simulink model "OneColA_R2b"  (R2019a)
settings: Solver=ode15s  StartTime=0.0  StopTime=tend  RelTol=1e-3
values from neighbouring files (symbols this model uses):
  alpha_L = -abs(alpha(2))    [TuningSRC.m]
  alpha_V = abs(alpha(1))    [TuningSRC.m]
  biasL = 3.2    [TuningSRC.m]
  biasV = VB0    [TuningSRC.m]
  DeltaxDmin = -0.01    [Simulate1Col_R2.m]
  Extract_J = zeros(83,1)'    [Simulate1Col.m]    (also in Simulate1Col_OL.m; Simulate1Col_R1.m; Simulate1Col_R2.m)
  Extract_xB = zeros(82,1)'    [Simulate1Col.m]    (also in Simulate1Col_OL.m; Simulate1Col_R1.m; Simulate1Col_R2.m)
  Extract_xD = zeros(82,1)'    [Simulate1Col.m]    (also in Simulate1Col_OL.m; Simulate1Col_R1.m; Simulate1Col_R2.m)
  F0 = 1    [colamod.m]    (also in ColumnA_simulation.m; Simulate1Col.m = F; Simulate1Col_OL.m = F; Simulate1Col_R1.m = F)
  F0step = 0.05    [Simulate1Col.m]    (also in Simulate1Col_OL.m = 1*F0*.1; Simulate1Col_R1.m; Simulate1Col_R2.m = 0.15)
  F0step2 = 0*(0.15-F0step)    (= 0)    [Simulate1Col.m]    (also in Simulate1Col_R1.m; Simulate1Col_R2.m = 0.1)
  F0step2_t = 30    [Simulate1Col.m]    (also in Simulate1Col_R1.m; Simulate1Col_R2.m = 80)
  F0step3 = 0    [Simulate1Col_R2.m]
  F0step3_t = 180    [Simulate1Col_R2.m]
  F0step_t = 10    [Simulate1Col.m]    (also in Simulate1Col_OL.m; Simulate1Col_R1.m; Simulate1Col_R2.m)
  Fbias = Fmax    (= 1.6825)    [Simulate1Col_R2.m]
  Fmax = 1.6825    [Simulate1Col_R2.m]
  Jcol = pf*u_all(5) + pV*u_all(2) - pB*u_all(4) - pD*u_all(3)    [ColumnA_simulation.m]    (also in col_obj.m = pf*F + pV*V - pB*B - pD*D; LVMassBalance.m = pf*Feed + pV*Steam - pB*B - pD*D)
  Kc_FxD = tau_FxD /(K_FxD *(tauc_FxD+theta_FxD))    (= -1.50442477876)    [TuningCol.m]
  Kc_LTxD = tau_LTxD /(K_LTxD *(tauc_LTxD+theta_LTxD))    (= 23.0752764867)    [TuningCol.m]
  Kc_SRC = abs(Kc_SRC)    [TuningSRC.m]
  KI_FxD = Kc_FxD/tauI_FxD    [TuningCol.m]
  KI_LTxD = Kc_LTxD/tauI_LTxD    [TuningCol.m]
  KI_SRC = Kc_SRC/tauI_SRC    [TuningSRC.m]
  LmaxPI = Lmax-LT0    [Simulate1Col.m]    (also in Simulate1Col_R1.m; Simulate1Col_R2.m)
  LT0 = u_opt(1)    [Simulate1Col.m]    (also in Simulate1Col_OL.m; Simulate1Col_R1.m; Simulate1Col_R2.m)
  pV0 = pV    [Simulate1Col.m]    (also in Simulate1Col_OL.m; Simulate1Col_R1.m; Simulate1Col_R2.m)
  pVstep = 0.02    [Simulate1Col.m]    (also in Simulate1Col_OL.m = 0*(0.13-pV0); Simulate1Col_R1.m; Simulate1Col_R2.m = 0.06)
  pVstep2 = 0    [Simulate1Col_R2.m]
  pVstep2t = 140    [Simulate1Col_R2.m]
  pVstept = 50    [Simulate1Col.m]    (also in Simulate1Col_OL.m; Simulate1Col_R1.m; Simulate1Col_R2.m)
  qF = U(7)    [colamod.m]    (also in ColumnA_simulation.m; Simulate1Col.m = 1; Simulate1Col_OL.m = 1; Simulate1Col_R1.m = 1)
  tauI_SRC = (tauI_VxB+tauI_LTxB)/2    [TuningSRC.m]
  VB0 = u_opt(2)    [Simulate1Col.m]    (also in Simulate1Col_OL.m; Simulate1Col_R1.m; Simulate1Col_R2.m)
  Vmax = 4    [Simulate1Col.m]    (also in Simulate1Col_R1.m; Simulate1Col_R2.m; TuningSRC.m)
  x0 = 0.5*ones(1,82)'    [col_obj.m]    (also in Simulate1Col.m = x; Simulate1Col_OL.m = x; Simulate1Col_R1.m = x; Simulate1Col_R2.m = x)
  xBsp = 0.95    [Simulate1Col.m]    (also in Simulate1Col_OL.m; Simulate1Col_R1.m; Simulate1Col_R2.m)
  xDmin = 0.95    [Simulate1Col.m]    (also in Simulate1Col_OL.m; Simulate1Col_R1.m; Simulate1Col_R2.m)
  zF = U(6)    [colamod.m]    (also in ColumnA_simulation.m; Simulate1Col.m = 0.5; Simulate1Col_OL.m = 0.5; Simulate1Col_R1.m = 0.5)
undefined symbols (not defined in the file or in its folder): Calc_xDsp, ColumnA_simulation, extract, LVMassBalance, SR_block
libraries: simulink x3

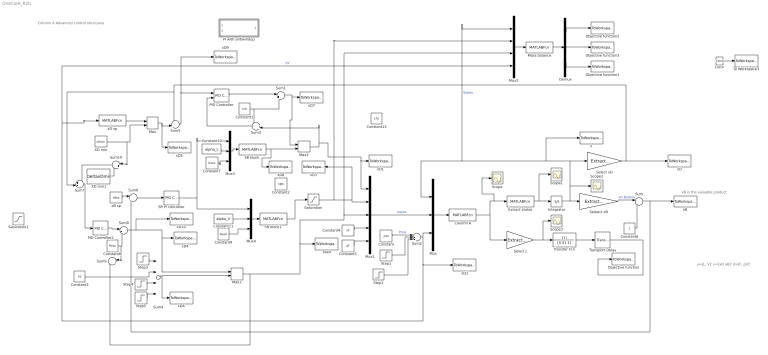
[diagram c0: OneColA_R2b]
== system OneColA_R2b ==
  note: u=[L, V]' y=[xD xB]' d=[F, pV]'
  note: xB is the valuable product
  note: Column A Advanced control structures
  Clock : Clock
  Column A : MATLABFcn  MATLABFcn=ColumnA_simulation(u)  OutputDimensions=83
  Constant : Constant  Value=pV0
  Constant1 : Constant  Value=LT0
  Constant10 : Constant  Value=alpha_L
  Constant11 : Constant  Value=alpha_V
  Constant13 : Constant  Value=LT0
  Constant2 : Constant  Value=VB0
  Constant3 : Constant  Value=F0
  Constant4 : Constant  Value=zF
  Constant5 : Constant  Value=qF
  Constant6 : Constant
  Constant7 : Constant  Value=biasL
  Constant8 : Constant  Value=Fbias
  Constant9 : Constant  Value=biasV
  Demux : Demux  Outputs=3
  Extract states : MATLABFcn  MATLABFcn=extract(u)  OutputDimensions=82
  Feed : ToWorkspace  VariableName=Fin  SampleTime=-1
  Integrator : Integrator  InitialCondition=x0
  Mass balance : MATLABFcn  MATLABFcn=LVMassBalance(u)  OutputDimensions=3
  Max : MinMax  Function=max  Inputs=2
  Max1 : MinMax  Inputs=2
  Max2 : MinMax  Inputs=2
  Mux : Mux  Inputs=3
  Mux1 : Mux  Inputs=5
  Mux2 : Mux
  Mux3 : Mux  Inputs=3
  Mux4 : Mux  Inputs=3
  Objective function : ToWorkspace  VariableName=Jactual  SampleTime=-1
  Objective function1 : ToWorkspace  VariableName=Jreal  SampleTime=-1
  Objective function2 : ToWorkspace  VariableName=Dcurrent  SampleTime=-1
  Objective function3 : ToWorkspace  VariableName=Bcurrent  SampleTime=-1
  PI with antiwindup : Subsystem
  PID Controller : simulink/Continuous/PID Controller  Controller=PI  Form=Parallel  TimeDomain=Continuous-time  SampleTime=-1  IntegratorMethod=Forward Euler  FilterMethod=Forward Euler  ControllerParametersSource=internal  P=Kc_LTxD  I=KI_LTxD  D=0  UseFilter=on  N=100  TunerSelectOption=Transfer Function Based (PID Tuner App)  InitialConditionSource=internal  InitialConditionForIntegrator=0  InitialConditionForFilter=0  DifferentiatorICPrevScaledInput=0  ExternalReset=none  TrackingMode=on  Kt=1  LimitOutput=on  UpperSaturationLimit=LmaxPI  LowerSaturationLimit=-LT0  LinearizeAsGain=on  AntiWindupMode=none  Kb=1  POutMin=[]  POutMax=[]  IOutMin=[]  IOutMax=[]  DOutMin=[]  DOutMax=[]  NOutMin=[]  NOutMax=[]  SumOutMin=[]  SumOutMax=[]  SaturationOutMin=[]  SaturationOutMax=[]  PParamMin=[]  PParamMax=[]  IParamMin=[]  IParamMax=[]  DParamMin=[]  DParamMax=[]  NParamMin=[]  NParamMax=[]  KbParamMin=[]  KbParamMax=[]  KtParamMin=[]  KtParamMax=[]  KbOutMin=[]  KbOutMax=[]  KtOutMin=[]  KtOutMax=[]  IntegratorOutMin=[]  IntegratorOutMax=[]  FilterOutMin=[]  FilterOutMax=[]  SumI1OutMin=[]  SumI1OutMax=[]  SumI2OutMin=[]  SumI2OutMax=[]  SumI3OutMin=[]  SumI3OutMax=[]  SumI4OutMin=[]  SumI4OutMax=[]  SumDOutMin=[]  SumDOutMax=[]  DifferentiatorOutMin=[]  DifferentiatorOutMax=[]  FilterDiffOutCoefMin=[]  FilterDiffOutCoefMax=[]  ReciprocalOutMin=[]  ReciprocalOutMax=[]  SumDenOutMin=[]  SumDenOutMax=[]  SumNumOutMin=[]  SumNumOutMax=[]  DivideOutMin=[]  DivideOutMax=[]  IntegratorContinuousStateAttributes=''  IntegratorStateMustResolveToSignalObject=off  IntegratorRTWStateStorageClass=Auto  FilterContinuousStateAttributes=''  FilterStateMustResolveToSignalObject=off  FilterRTWStateStorageClass=Auto  ParallelPVariant=InternalParameters  IdealPVariant=Disabled  IVariant=InternalParameters  DVariant=Disabled  IntegratorVariant=Continuous  SatVariant=Enabled  AWVariant=Passthrough  PCopyVariant=Disabled  TRVariant=Enabled  FdbkBlocksVariant=Forward  IdealPFdbkVariant=Disabled  SatFdbkVariant=Disabled  DerivativeFilterVariant=Disabled  NVariant=Disabled  NCopyVariant=Disabled_SignalSpec  FilterICVariant=Disabled  IntegratorICVariant=InternalICs  ExternalResetVariant=Disabled  TRSumVariant=TrackingMode  SumFdbkVariant=Disabled  SumVariant=Sum_PI
  PID Controller2 : simulink/Continuous/PID Controller  Controller=P  Form=Parallel  TimeDomain=Continuous-time  SampleTime=-1  IntegratorMethod=Forward Euler  FilterMethod=Forward Euler  ControllerParametersSource=internal  P=Kc_FxD  I=KI_FxD  D=0  UseFilter=on  N=100  TunerSelectOption=Transfer Function Based (PID Tuner App)  InitialConditionSource=internal  InitialConditionForIntegrator=0  InitialConditionForFilter=0  DifferentiatorICPrevScaledInput=0  ExternalReset=none  TrackingMode=on  Kt=1  LimitOutput=on  UpperSaturationLimit=inf  LowerSaturationLimit=-inf  LinearizeAsGain=on  AntiWindupMode=none  Kb=1  POutMin=[]  POutMax=[]  IOutMin=[]  IOutMax=[]  DOutMin=[]  DOutMax=[]  NOutMin=[]  NOutMax=[]  SumOutMin=[]  SumOutMax=[]  SaturationOutMin=[]  SaturationOutMax=[]  PParamMin=[]  PParamMax=[]  IParamMin=[]  IParamMax=[]  DParamMin=[]  DParamMax=[]  NParamMin=[]  NParamMax=[]  KbParamMin=[]  KbParamMax=[]  KtParamMin=[]  KtParamMax=[]  KbOutMin=[]  KbOutMax=[]  KtOutMin=[]  KtOutMax=[]  IntegratorOutMin=[]  IntegratorOutMax=[]  FilterOutMin=[]  FilterOutMax=[]  SumI1OutMin=[]  SumI1OutMax=[]  SumI2OutMin=[]  SumI2OutMax=[]  SumI3OutMin=[]  SumI3OutMax=[]  SumI4OutMin=[]  SumI4OutMax=[]  SumDOutMin=[]  SumDOutMax=[]  DifferentiatorOutMin=[]  DifferentiatorOutMax=[]  FilterDiffOutCoefMin=[]  FilterDiffOutCoefMax=[]  ReciprocalOutMin=[]  ReciprocalOutMax=[]  SumDenOutMin=[]  SumDenOutMax=[]  SumNumOutMin=[]  SumNumOutMax=[]  DivideOutMin=[]  DivideOutMax=[]  IntegratorContinuousStateAttributes=''  IntegratorStateMustResolveToSignalObject=off  IntegratorRTWStateStorageClass=Auto  FilterContinuousStateAttributes=''  FilterStateMustResolveToSignalObject=off  FilterRTWStateStorageClass=Auto  ParallelPVariant=InternalParameters  IdealPVariant=Disabled  IVariant=Disabled  DVariant=Disabled  IntegratorVariant=Disabled  SatVariant=Enabled  AWVariant=Disabled  PCopyVariant=Disabled  TRVariant=Disabled  FdbkBlocksVariant=Forward  IdealPFdbkVariant=Disabled  SatFdbkVariant=Disabled  DerivativeFilterVariant=Disabled  NVariant=Disabled  NCopyVariant=Disabled_SignalSpec  FilterICVariant=Disabled  IntegratorICVariant=Disabled  ExternalResetVariant=Disabled  TRSumVariant=Passthrough  SumFdbkVariant=Disabled  SumVariant=Passthrough_P
  SR PI controller : simulink/Continuous/PID Controller  Controller=PI  Form=Parallel  TimeDomain=Continuous-time  SampleTime=-1  IntegratorMethod=Forward Euler  FilterMethod=Forward Euler  ControllerParametersSource=internal  P=Kc_SRC  I=KI_SRC  D=0  UseFilter=on  N=100  TunerSelectOption=Transfer Function Based (PID Tuner App)  InitialConditionSource=internal  InitialConditionForIntegrator=0  InitialConditionForFilter=0  DifferentiatorICPrevScaledInput=0  ExternalReset=none  TrackingMode=off  Kt=1  LimitOutput=on  UpperSaturationLimit=inf  LowerSaturationLimit=-inf  LinearizeAsGain=on  AntiWindupMode=none  Kb=1  POutMin=[]  POutMax=[]  IOutMin=[]  IOutMax=[]  DOutMin=[]  DOutMax=[]  NOutMin=[]  NOutMax=[]  SumOutMin=[]  SumOutMax=[]  SaturationOutMin=[]  SaturationOutMax=[]  PParamMin=[]  PParamMax=[]  IParamMin=[]  IParamMax=[]  DParamMin=[]  DParamMax=[]  NParamMin=[]  NParamMax=[]  KbParamMin=[]  KbParamMax=[]  KtParamMin=[]  KtParamMax=[]  KbOutMin=[]  KbOutMax=[]  KtOutMin=[]  KtOutMax=[]  IntegratorOutMin=[]  IntegratorOutMax=[]  FilterOutMin=[]  FilterOutMax=[]  SumI1OutMin=[]  SumI1OutMax=[]  SumI2OutMin=[]  SumI2OutMax=[]  SumI3OutMin=[]  SumI3OutMax=[]  SumI4OutMin=[]  SumI4OutMax=[]  SumDOutMin=[]  SumDOutMax=[]  DifferentiatorOutMin=[]  DifferentiatorOutMax=[]  FilterDiffOutCoefMin=[]  FilterDiffOutCoefMax=[]  ReciprocalOutMin=[]  ReciprocalOutMax=[]  SumDenOutMin=[]  SumDenOutMax=[]  SumNumOutMin=[]  SumNumOutMax=[]  DivideOutMin=[]  DivideOutMax=[]  IntegratorContinuousStateAttributes=''  IntegratorStateMustResolveToSignalObject=off  IntegratorRTWStateStorageClass=Auto  FilterContinuousStateAttributes=''  FilterStateMustResolveToSignalObject=off  FilterRTWStateStorageClass=Auto  ParallelPVariant=InternalParameters  IdealPVariant=Disabled  IVariant=InternalParameters  DVariant=Disabled  IntegratorVariant=Continuous  SatVariant=Enabled  AWVariant=Passthrough  PCopyVariant=Disabled  TRVariant=Disabled  FdbkBlocksVariant=Forward  IdealPFdbkVariant=Disabled  SatFdbkVariant=Disabled  DerivativeFilterVariant=Disabled  NVariant=Disabled  NCopyVariant=Disabled_SignalSpec  FilterICVariant=Disabled  IntegratorICVariant=InternalICs  ExternalResetVariant=Disabled  TRSumVariant=Passthrough  SumFdbkVariant=Disabled  SumVariant=Sum_PI
  SR block : MATLABFcn  MATLABFcn=SR_block(u)  OutputDimensions=1
  SR block1 : MATLABFcn  MATLABFcn=SR_block(u)  OutputDimensions=1
  Saturation : Saturate  UpperLimit=Vmax  LowerLimit=0
  Saturation1 : Saturate  UpperLimit=Fmax  LowerLimit=1
  Scope{,1..3} (4 alike) : Scope
  Select J : Gain  Gain=Extract_J  Multiplication=Matrix(K*u)
  Select xD : Gain  Gain=Extract_xD  Multiplication=Matrix(K*u)
  Seleect xB : Gain  Gain=Extract_xB  Multiplication=Matrix(K*u)
  Step1 : Step  Time=pVstept  After=pVstep  SampleTime=0
  Step2 : Step  Time=pVstep2t  After=pVstep2  SampleTime=0
  Step3 : Step  Time=F0step_t  After=F0step  SampleTime=0
  Step4 : Step  Time=F0step2_t  After=F0step2  SampleTime=0
  Step5 : Step  Time=F0step3_t  After=F0step3  SampleTime=0
  Sum : Sum  Inputs=|-+
  Sum1 : Sum  Inputs=|++
  Sum10 : Sum  Inputs=|++
  Sum2 : Sum  Inputs=|+++
  Sum3 : Sum  Inputs=-+|
  Sum4 : Sum  Inputs=++++
  Sum5 : Sum  Inputs=-+|
  Sum6 : Sum  Inputs=|+-
  Sum7 : Sum  Inputs=+-|
  Sum8 : Sum  Inputs=|++
  Sum9 : Sum  Inputs=|-+
  To Workspace3 : ToWorkspace  VariableName=time  SampleTime=-1
  Transfer Fcn : TransferFcn  Denominator=[0.01 1]
  Transport Delay : TransportDelay  DelayTime=0.5  InitialOutput=Jcol
  XD min : Constant  Value=xDmin
  XD min1 : Constant  Value=DeltaxDmin
  x : ToWorkspace  VariableName=States  SampleTime=-1
  xB : ToWorkspace  VariableName=xB  SampleTime=-1
  xB sp : Constant  Value=xBsp
  xD : ToWorkspace  VariableName=xD  SampleTime=-1
  xD sp : MATLABFcn  MATLABFcn=Calc_xDsp(u)  OutputDimensions=1
  xD1 : ToWorkspace  VariableName=LT  SampleTime=-1
  xD10 : ToWorkspace  VariableName=Fin_xD1  SampleTime=-1
  xD2 : ToWorkspace  VariableName=pV  SampleTime=-1
  xD3 : ToWorkspace  VariableName=VB  SampleTime=-1
  xD4 : ToWorkspace  VariableName=Fin_xD  SampleTime=-1
  xD5 : ToWorkspace  VariableName=xDsp  SampleTime=-1
  xD6 : ToWorkspace  VariableName=Fin_sp  SampleTime=-1
  xD7 : ToWorkspace  VariableName=LTxD  SampleTime=-1
  xD8 : ToWorkspace  VariableName=LTSR  SampleTime=-1
  xD9 : ToWorkspace  VariableName=error_xD  SampleTime=-1
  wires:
  Mux/1 -> Column A/1
  Mux1/1 -> Mux/2  "Inputs"
  Constant4/1 -> Mux1/4
  Constant5/1 -> Mux1/5
  Column A/1 -> Select J/1, Extract states/1, Scope/1
  Extract states/1 -> Scope1/1, Integrator/1
  Integrator/1 -> Seleect xB/1, Select xD/1, x/1, Mux2/1, Mux/1, Scope2/1  "States"
  Select xD/1 -> Sum5/1, Sum7/2, xD/1
  Select J/1 -> Scope3/1, Transfer Fcn/1
  Clock/1 -> To Workspace3/1
  Seleect xB/1 -> Sum/1  "xD Bottom"
  Sum/1 -> xB/1, Sum6/2
  Constant6/1 -> Sum/2
  Sum2/1 -> xD2/1, xD sp/1, Mux2/4, Mux/3  "pV"
  Constant/1 -> Sum2/1  "Price"
  Step1/1 -> Sum2/2
  Sum6/1 -> SR PI controller/1
  xB sp/1 -> Sum6/1
  Max/1 -> xD5/1, Sum5/2
  xD sp/1 -> Max/1
  XD min/1 -> Sum10/1, Max/2
  Constant3/1 -> Sum4/2
  Step4/1 -> Sum4/3
  Step3/1 -> Sum4/1
  Max1/1 -> Mux2/3, Mux1/3, Feed/1, Sum9/2
  Sum7/1 -> PID Controller2/1
  Sum4/1 -> Max1/2, xD6/1
  PID Controller2/1 -> Sum8/1
  Constant8/1 -> Sum9/1, Sum8/2
  Mass balance/1 -> Demux/1
  Demux/3 -> Objective function1/1
  Mux2/1 -> Mass balance/1
  Demux/1 -> Objective function2/1
  Demux/2 -> Objective function3/1
  SR block/1 -> xD8/1, Max2/2
  Mux3/1 -> SR block/1
  Mux4/1 -> SR block1/1
  SR PI controller/1 -> Mux3/1, Mux4/1
  Constant7/1 -> Mux3/3
  Constant9/1 -> Mux4/3
  Constant10/1 -> Mux3/2
  Constant11/1 -> Mux4/2
  Saturation/1 -> Mux1/2, xD3/1, Mux2/2
  Sum1/1 -> Max2/1, xD7/1
  Max2/1 -> xD1/1, Mux1/1, Sum3/2
  SR block1/1 -> Saturation/1
  Sum5/1 -> PID Controller/1, xD9/1
  PID Controller/1 -> Sum1/1
  Constant1/1 -> Sum3/1, Sum1/2
  Sum3/1 -> PID Controller/2
  Step2/1 -> Sum2/3
  Transport Delay/1 -> Objective function/1
  Transfer Fcn/1 -> Transport Delay/1
  Step5/1 -> Sum4/4
  Sum8/1 -> Max1/1, xD4/1, xD10/1
  Sum10/1 -> Sum7/1
  XD min1/1 -> Sum10/2

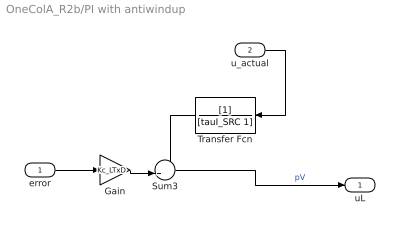
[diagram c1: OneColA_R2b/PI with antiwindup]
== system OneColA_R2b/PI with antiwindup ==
  error : Inport
  u_actual : Inport  Port=2
  Gain : Gain  Gain=Kc_LTxD
  Sum3 : Sum  Inputs=++|
  Transfer Fcn : TransferFcn  Denominator=[tauI_SRC 1]
  uL : Outport
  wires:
  Transfer Fcn/1 -> Sum3/1
  Gain/1 -> Sum3/2
  Sum3/1 -> uL/1  "pV"
  u_actual/1 -> Transfer Fcn/1
  error/1 -> Gain/1
